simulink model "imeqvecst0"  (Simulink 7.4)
settings: Solver=ode45  StartTime=0.0  StopTime=3  MaxStep=2e-4  RelTol=1e-3

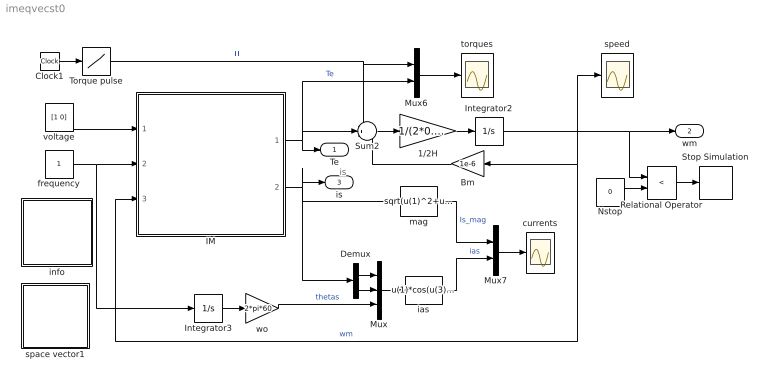
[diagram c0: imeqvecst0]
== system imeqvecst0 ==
  note: is
  1/2H : Gain  Gain=1/(2*0.3)  ParameterDataType=sfix(16)  ParameterScaling=2^0  OutDataType=sfix(16)  OutScaling=2^0
  Bm : Gain  Gain=1e-6  ParameterDataType=sfix(16)  ParameterScaling=2^0  OutDataType=sfix(16)  OutScaling=2^0
  Clock1 : Clock
  Demux : Demux  Outputs=2
  IM : Subsystem  mask(Inductionmachine){Rs=0.01, Rr=0.02, Lsl=0.10, Lrl=0.10, Lm=4.50, wo=2*pi*60}
      mask prompts: Rs "Stator resistance [pu]"; Rr "Rotor resistance [pu]"; Lsl "Stator leakage inductance [pu]"; Lrl "Rotor leakage inductance [pu]"; Lm "Magnetizing inductance [pu]"; wo "Base frequency [rad/s]"
      mask help: Induction motor subsystem model using state space formulation in an arbitrary reference frame k. Parameters are expressed in per unit.
  Integrator2 : Integrator
  Integrator3 : Integrator
  Mux : Mux  Inputs=3
  Mux6 : Mux  Inputs=2
  Mux7 : Mux  Inputs=2
  Nstop : Constant  Value=0  OutDataType=sfix(16)  OutScaling=2^0
  Relational Operator : RelationalOperator  Operator=<
  Stop Simulation : Stop
  Sum2 : Sum  Inputs=-+-  OutDataType=sfix(16)  OutScaling=2^0
  Torque pulse : Lookup  InputValues=[0 1.4 3 ]  Table="[0  0  4 ]"  OutDataType=sfix(16)  OutScaling=2^0
  currents : Scope
  frequency : Constant  OutDataType=sfix(16)  OutScaling=2^0
  ias : Fcn  Expr=u(1)*cos(u(3))-u(2)*sin(u(3))
  info : Subsystem
  mag : Fcn  Expr=sqrt(u(1)^2+u(2)^2)
  space vector1 : Subsystem
  speed : Scope
  torques : Scope
  voltage : Constant  Value=[1 0]  OutDataType=sfix(16)  OutScaling=2^0
  wo : Gain  Gain=2*pi*60  ParameterDataType=sfix(16)  ParameterScaling=2^0  OutDataType=sfix(16)  OutScaling=2^0
  Te : Outport
  wm : Outport  Port=2
  is : Outport  Port=3
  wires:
  voltage/1 -> IM/1(vs)
  frequency/1 -> Integrator3/1, IM/2(wk)
  Demux/1 -> Mux/1
  Demux/2 -> Mux/2
  Mux/1 -> ias/1
  ias/1 -> Mux7/2  "ias"
  mag/1 -> Mux7/1  "Is_mag"
  Mux7/1 -> currents/1
  Sum2/1 -> 1/2H/1
  1/2H/1 -> Integrator2/1
  Clock1/1 -> Torque pulse/1
  Torque pulse/1 -> Mux6/1, Sum2/1  "Tl"
  Integrator3/1 -> wo/1
  wo/1 -> Mux/3  "thetas"
  Mux6/1 -> torques/1
  Bm/1 -> Sum2/3
  Integrator2/1 -> IM/3(wm), Bm/1, speed/1, wm/1, Relational Operator/1  "wm"
  IM/1(Te) -> Sum2/2, Mux6/2, Te/1  "Te"
  IM/2(is) -> mag/1, Demux/1, is/1
  Nstop/1 -> Relational Operator/2
  Relational Operator/1 -> Stop Simulation/1

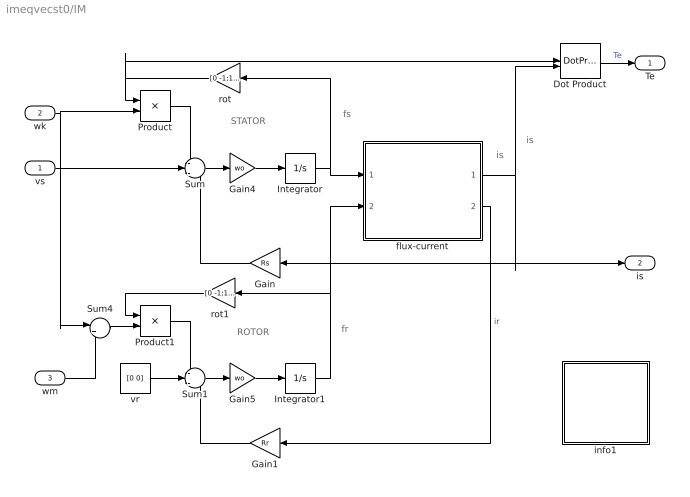
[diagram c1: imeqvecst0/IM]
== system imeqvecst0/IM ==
  note: ROTOR
  note: STATOR
  note: fs
  note: fr
  note: is
  note: is
  vs : Inport  OutDataType=sfix(16)  OutScaling=2^0
  wk : Inport  Port=2  OutDataType=sfix(16)  OutScaling=2^0
  wm : Inport  Port=3  OutDataType=sfix(16)  OutScaling=2^0
  Dot Product : DotProduct  OutDataType=fixdt(1, 16)  OutScaling=2^-10
  Gain : Gain  Gain=Rs  ParameterDataType=sfix(16)  ParameterScaling=2^0  OutDataType=sfix(16)  OutScaling=2^0
  Gain1 : Gain  Gain=Rr  ParameterDataType=sfix(16)  ParameterScaling=2^0  OutDataType=sfix(16)  OutScaling=2^0
  Gain4 : Gain  Gain=wo  ParameterDataType=sfix(16)  ParameterScaling=2^0  OutDataType=sfix(16)  OutScaling=2^0
  Gain5 : Gain  Gain=wo  ParameterDataType=sfix(16)  ParameterScaling=2^0  OutDataType=sfix(16)  OutScaling=2^0
  Integrator : Integrator  InitialCondition=[0 0]
  Integrator1 : Integrator  InitialCondition=[0 0]
  Product : Product  OutDataType=sfix(16)  OutScaling=2^0
  Product1 : Product  OutDataType=sfix(16)  OutScaling=2^0
  Sum : Sum  Inputs=-+-  OutDataType=sfix(16)  OutScaling=2^0
  Sum1 : Sum  Inputs=-+-  OutDataType=sfix(16)  OutScaling=2^0
  Sum4 : Sum  Inputs=|+-  OutDataType=sfix(16)  OutScaling=2^0
  flux-current : Subsystem
  info1 : Subsystem
  rot : Gain  Gain=[0 -1;1 0]  Multiplication=Matrix(K*u)  ParameterDataType=sfix(16)  ParameterScaling=2^0  OutDataType=sfix(16)  OutScaling=2^0
  rot1 : Gain  Gain=[0 -1;1 0]  Multiplication=Matrix(K*u)  ParameterDataType=sfix(16)  ParameterScaling=2^0  OutDataType=sfix(16)  OutScaling=2^0
  vr : Constant  Value=[0 0]  OutDataType=sfix(16)  OutScaling=2^0
  Te : Outport
  is : Outport  Port=2
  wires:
  Gain/1 -> Sum/3
  vr/1 -> Sum1/2
  Gain1/1 -> Sum1/3
  flux-current/2(ir) -> Gain1/1  "ir"
  Integrator/1 -> flux-current/1(fs), rot/1
  Integrator1/1 -> rot1/1, flux-current/2(fr)
  Product1/1 -> Sum1/1
  rot1/1 -> Product1/1
  Product/1 -> Sum/1
  rot/1 -> Product/1, Dot Product/1
  Sum4/1 -> Product1/2
  Sum/1 -> Gain4/1
  Gain4/1 -> Integrator/1
  Sum1/1 -> Gain5/1
  Gain5/1 -> Integrator1/1
  flux-current/1(is) -> Gain/1, is/1, Dot Product/2
  Dot Product/1 -> Te/1  "Te"
  vs/1 -> Sum/2
  wk/1 -> Product/2, Sum4/1
  wm/1 -> Sum4/2

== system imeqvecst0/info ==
  note: Starting of an induction motor
  note: This demonstration illustrates the line starting of an induction motor at no load followed by ramping the load torque. You will thus be able to compare the torque-speed characteristics of the machine under both dynamic and quasi-steady state conditions. To modify the machine parameters, double click the induction motor block.

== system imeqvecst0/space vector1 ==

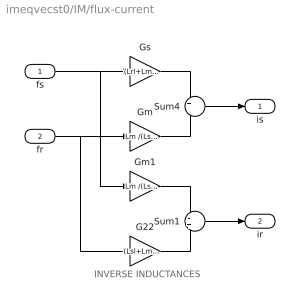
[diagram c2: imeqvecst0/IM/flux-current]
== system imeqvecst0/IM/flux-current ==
  note: INVERSE INDUCTANCES
  fs : Inport  OutDataType=sfix(16)  OutScaling=2^0
  fr : Inport  Port=2  OutDataType=sfix(16)  OutScaling=2^0
  G22 : Gain  Gain=(Lsl+Lm )/(Lsl*Lrl+Lsl*Lm+Lrl*Lm)  ParameterDataType=sfix(16)  ParameterScaling=2^0  OutDataType=sfix(16)  OutScaling=2^0
  Gm : Gain  Gain=Lm /(Lsl*Lrl+Lsl*Lm+Lrl*Lm)  ParameterDataType=sfix(16)  ParameterScaling=2^0  OutDataType=sfix(16)  OutScaling=2^0
  Gm1 : Gain  Gain=Lm /(Lsl*Lrl+Lsl*Lm+Lrl*Lm)  ParameterDataType=sfix(16)  ParameterScaling=2^0  OutDataType=sfix(16)  OutScaling=2^0
  Gs : Gain  Gain=(Lrl+Lm) /(Lsl*Lrl+Lsl*Lm+Lrl*Lm)  ParameterDataType=sfix(16)  ParameterScaling=2^0  OutDataType=sfix(16)  OutScaling=2^0
  Sum1 : Sum  Inputs=-+  OutDataType=sfix(16)  OutScaling=2^0
  Sum4 : Sum  Inputs=+-  OutDataType=sfix(16)  OutScaling=2^0
  is : Outport
  ir : Outport  Port=2
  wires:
  fs/1 -> Gs/1, Gm1/1
  Gs/1 -> Sum4/1
  fr/1 -> Gm/1, G22/1
  Gm/1 -> Sum4/2
  Sum4/1 -> is/1
  Gm1/1 -> Sum1/1
  G22/1 -> Sum1/2
  Sum1/1 -> ir/1

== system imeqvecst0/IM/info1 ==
  note: This demonstration illustrates the dynamics of a synchronous generator, initially at no load, following a three-phase short circuit at the terminals.
  note: Synchronous machine transients under shortcircuit
